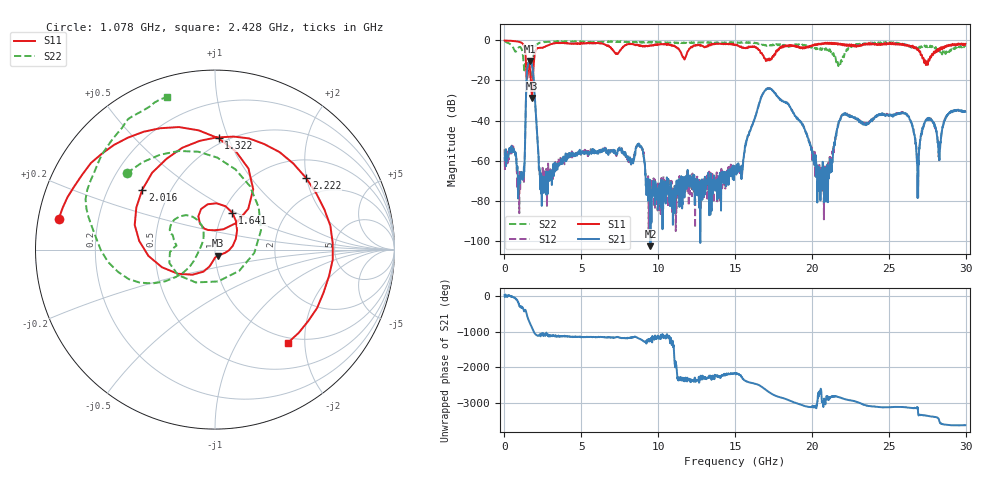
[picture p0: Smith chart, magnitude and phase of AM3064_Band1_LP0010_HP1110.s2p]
# Hz S DB R 50.0
!freq dBS11 angS11 dBS21 angS21 dBS12 angS12 dBS22 angS22
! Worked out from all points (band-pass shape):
!   1600 points, 10 MHz to 29.98 GHz, reference 50 ohm
!   highest |S21| = -10.26 dB at 1.678 GHz (marker M1); lowest = -102.8 dB at 9.494 GHz (marker M2)
!   |S21| within 3 dB of the highest: 1.502 GHz to 1.816 GHz (313.9 MHz wide, 18.9 % of centre)
!   lowest |S11| = -28.8 dB at 1.791 GHz (marker M3), VSWR 1.08, Z = 51.4 - j3.44 ohm
!   |S11| at or under -10 dB: 1.392 GHz to 1.923 GHz (531.1 MHz wide, 32 % of centre); 27.27982 GHz to 27.35189 GHz (72.07 MHz wide, 0.264 % of centre); 27.36 GHz to 27.57 GHz (206.9 MHz wide, 0.753 % of centre)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
!   |S22| runs from -22.0 to -0.3 dB; largest |S21 - S12| = 0.0059
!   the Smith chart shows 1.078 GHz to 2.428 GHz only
!   S11 on the Smith chart (normalised r, x): 1.078 GHz: 0.06, +0.10; 1.322 GHz: 0.46, +0.92; 1.641 GHz: 1.11, +0.48; 2.016 GHz: 0.35, +0.32; 2.222 GHz: 1.46, +1.99; 2.428 GHz: 0.91, -1.67
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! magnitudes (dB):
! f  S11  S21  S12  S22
! 10 MHz  0.0  -58.7  -54.4  -0.3
! 1.078 GHz  -1.0  -67.5  -65.9  -3.7
! 1.322 GHz  -4.1  -57.8  -57.2  -13.5
! 1.641 GHz  -12.9  -10.4  -10.4  -13.1
! 1.678 GHz  -15.7  -10.3  -10.3  -16.4
! 1.791 GHz  -28.8  -12.1  -12.1  -17.4
! 2.016 GHz  -5.6  -33.4  -33.3  -3.1
! 2.222 GHz  -3.8  -58.1  -57.3  -1.5
! 2.428 GHz  -3.6  -82.6  -68.0  -1.0
! 5.015 GHz  -1.5  -56.1  -56.2  -0.7
! 8.782 GHz  -2.6  -52.5  -52.1  -0.8
! 9.494 GHz  -2.5  -102.8  -70.0  -0.8
! 10 GHz  -2.0  -73.9  -74.7  -0.9
! 15 GHz  -2.3  -62.9  -65.6  -1.2
! 17.14 GHz  -10.0  -23.9  -23.9  -2.6
! 19.99 GHz  -2.9  -54.7  -53.9  -3.5
! 20.95 GHz  -1.7  -72.3  -63.4  -4.4
! 22.02 GHz  -2.5  -37.1  -37.2  -7.9
! 25 GHz  -1.4  -37.2  -37.1  -1.1
! 26.89 GHz  -4.4  -67.5  -75.0  -3.7
! 27.47 GHz  -10.5  -39.4  -39.1  -2.7
! 29.98 GHz  -1.7  -35.7  -35.5  -3.1
